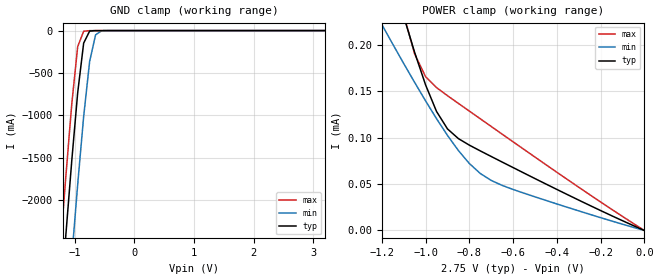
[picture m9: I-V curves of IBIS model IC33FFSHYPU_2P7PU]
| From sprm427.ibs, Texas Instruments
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|   Model IC33FFSHYPU_2P7PU
[Model]   IC33FFSHYPU_2P7PU
Model_type   Input
Polarity   Non-Inverting
Vinl =   0.8250V
Vinh =   1.9250V
C_comp   2.1397pF   2.1317pF   2.1767pF
[Temperature Range]   25.0000   0.1250k   -40.0000
[Voltage Range]   2.7500V   2.5000V   3.0000V
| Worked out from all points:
|   GND clamp passes 1 mA (typ) near -0.66 V on its own axis
|   POWER clamp passes 1 mA (typ) near -1.95 V on its own axis
[GND_clamp]
| voltage   I(typ)   I(min)   I(max)
-2.75V    -17.91A    -19.01A    -17.27A
-1.25V    -3.342A    -4.502A    -2.646A
-1.15V    -2.424A    -3.58A     -1.732A
-1.05V    -1.541A    -2.68A     -871.7mA
-950mV    -732.8mA   -1.814A    -188.7mA
-850mV    -147.9mA   -1.014A    -7.878mA
-750mV    -6.082mA   -364.9mA   -938.7uA
-650mV    -293.7uA   -49.99mA   -199.5uA
-550mV    -97.65uA   -3.277mA   -142.7uA
3.2V      0A         0A         0A
[POWER_clamp]
| voltage   I(typ)   I(min)   I(max)
-2.75V    1.763mA    922.7uA    2.451mA
-1.2V     314.6uA    222.2uA    344.7uA
-1.15V    272.1uA    201uA      286uA
-1.1V     231uA      180.1uA    232.7uA
-1.05V    192.1uA    159.7uA    190.4uA
-1V       157uA      139.8uA    165.9uA
-950mV    128.4uA    120.6uA    154.2uA
-900mV    109.6uA    102.6uA    145.4uA
-850mV    99.1uA     86.22uA    137.1uA
-750mV    85.86uA    61.49uA    120.5uA
-650mV    73.82uA    48.63uA    103.9uA
0V        176.2pA    1.233nA    189.2pA
